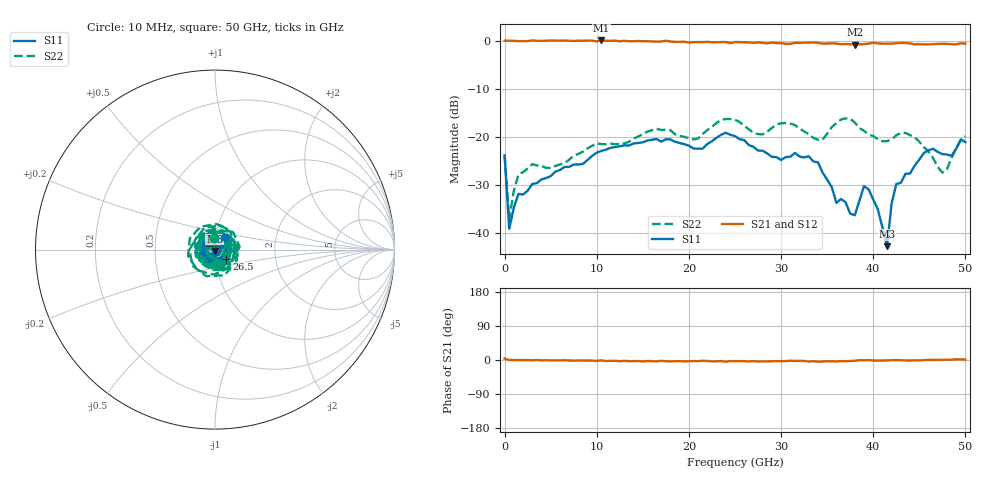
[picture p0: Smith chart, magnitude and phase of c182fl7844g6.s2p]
! 8/5/2019 2:58:39 PM
! Z:\MATT MILLER ENGINEERING\C182FL7844G6.S2P
! CHANNEL.1
! TR.MEASUREMENT
! CORRECTED.DATA
# GHZ S RI R 50.0
! FREQ.GHZ  S11RE  S11IM  S21RE  S21IM  S12RE  S12IM  S22RE  S22IM
!; PortSelection: Port_12
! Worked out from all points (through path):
!   101 points, 10 MHz to 50 GHz, reference 50 ohm
!   highest |S21| = 0.03 dB at 10.51 GHz (marker M1); lowest = -0.8 dB at 38 GHz (marker M2)
!   lowest |S11| = -42.7 dB at 41.5 GHz (marker M3), VSWR 1.01, Z = 49.9 - j0.731 ohm
!   |S11| at or under -10 dB: start of sweep to end of sweep
!   |S22| runs from -37.1 to -16.1 dB; largest |S21 - S12| = 0.036
!   S11 on the Smith chart (normalised r, x): 10 MHz: 0.98, +0.13; 26.5 GHz: 1.13, -0.12; 50 GHz: 1.10, +0.16
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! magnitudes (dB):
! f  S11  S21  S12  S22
! 10 MHz  -23.8  0.0  0.0  -23.8
! 509.9 MHz  -39.1  0.0  0.0  -37.1
! 1.51 GHz  -31.8  -0.1  -0.1  -27.8
! 8.508 GHz  -25.6  0.0  -0.1  -23.1
! 10.51 GHz  -22.9  0.0  0.0  -21.5
! 17.01 GHz  -21.0  -0.2  -0.1  -18.6
! 20.51 GHz  -22.4  -0.3  -0.3  -20.5
! 25 GHz  -19.8  -0.3  -0.3  -16.4
! 26.5 GHz  -21.7  -0.4  -0.5  -18.4
! 31 GHz  -24.1  -0.7  -0.6  -17.2
! 33.5 GHz  -25.1  -0.4  -0.4  -20.2
! 36 GHz  -33.7  -0.6  -0.7  -17.1
! 38 GHz  -36.2  -0.8  -0.7  -17.0
! 39 GHz  -30.2  -0.7  -0.7  -18.7
! 39.5 GHz  -30.9  -0.6  -0.6  -19.5
! 40.5 GHz  -35.0  -0.6  -0.7  -20.5
! 41.5 GHz  -42.7  -0.6  -0.6  -20.9
! 42 GHz  -33.7  -0.6  -0.6  -20.5
! 42.5 GHz  -29.8  -0.5  -0.6  -19.7
! 45.5 GHz  -23.3  -0.8  -0.7  -22.1
! 47.5 GHz  -23.5  -0.7  -0.6  -27.4
! 50 GHz  -21.1  -0.6  -0.6  -19.8
